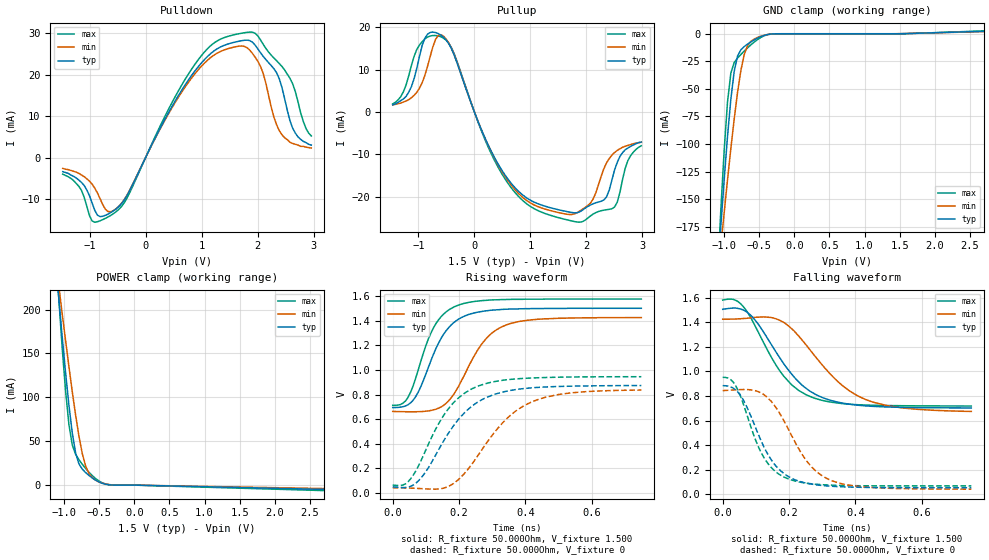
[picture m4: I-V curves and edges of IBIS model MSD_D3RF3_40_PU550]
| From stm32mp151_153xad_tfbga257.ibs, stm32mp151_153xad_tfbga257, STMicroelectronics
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[Model] MSD_D3RF3_40_PU550
Model_type   I/O
C_comp 2.417pF   2.334pF   2.540pF
Vinh = 925.000mV
Vinl = 575.000mV
Vmeas = 750.000mV
Vref = 750.000mV
[Model Spec]
Vinh   925.000mV   888.000mV   963.000mV
Vinl   575.000mV   538.000mV   613.000mV
Vmeas   750.000mV   713.000mV   788.000mV
Vref   750.000mV   713.000mV   788.000mV
[Temperature Range]   25.000   125.000   -40.000
[Voltage Range]   1.500V   1.425V   1.575V
[GND Clamp Reference]   0.00V   0.00V   0.00V
[Pulldown Reference]   0.00V   0.00V   0.00V
[POWER Clamp Reference]   1.500V   1.425V   1.575V
[Pullup Reference]   1.500V   1.425V   1.575V
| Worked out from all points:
|   slope of the pulldown table from 0 to 0.225 V, typ, clamps not added: 36.6 ohm
|   slope of the pullup table from 0 to 0.225 V, typ, clamps not added: 31.2 ohm
|   GND clamp passes 1 mA (typ) near -0.40 V on its own axis
|   POWER clamp passes 1 mA (typ) near -0.41 V on its own axis
|   rising waveform, R_fixture 50.000Ohm, V_fixture 1.500: 20-80 % time 84.3ps typ, 101ps min, 73.8ps max; typ from 0.694 V to 1.5 V
|   rising waveform, R_fixture 50.000Ohm, V_fixture 0: 20-80 % time 131ps typ, 148ps min, 115ps max; typ from 0.05 V to 0.873 V
|   falling waveform, R_fixture 50.000Ohm, V_fixture 1.500: 20-80 % time 134ps typ, 159ps min, 118ps max; typ from 1.5 V to 0.703 V
|   falling waveform, R_fixture 50.000Ohm, V_fixture 0: 20-80 % time 92.7ps typ, 110ps min, 81.1ps max; typ from 0.884 V to 0.055 V
[GND Clamp]
-1.48V    -594.8mA   -480.5mA   -764.4mA
-1.098V   -218.8mA   -223.8mA   -221mA
-1.05V    -174.6mA   -192.8mA   -160.3mA
-1.002V   -132.4mA   -162.4mA   -105.9mA
-954.6mV  -93.29mA   -132.7mA   -62.13mA
-906.8mV  -59.43mA   -104.2mA   -35.7mA
-859.1mV  -34.17mA   -77.46mA   -26.12mA
-811.4mV  -20.23mA   -53.34mA   -22.06mA
-715.9mV  -11.65mA   -18.94mA   -15.73mA
-572.7mV  -5.552mA   -4.746mA   -7.503mA
-286.4mV  -69.21uA   -117uA     -55.41uA
2.959V    2.671mA    2.278mA    3.222mA
[Power Clamp]
-1.459V   578.6mA    480mA      724.3mA
-1.077V   211.6mA    226mA      211.1mA
-1.03V    168.7mA    195.2mA    156.3mA
-981.8mV  128.1mA    164.8mA    107.4mA
-934.1mV  90.98mA    135.1mA    68.88mA
-886.4mV  59.46mA    106.6mA    45.73mA
-838.6mV  36.57mA    79.76mA    35.11mA
-743.2mV  18.16mA    35.82mA    23.68mA
-647.7mV  10.96mA    13.03mA    14.61mA
-552.3mV  5.616mA    5.561mA    7.395mA
-313.6mV  108.4uA    247.8uA    122.3uA
2.98V     -5.382mA   -4.337mA   -6.867mA
[Pulldown]
-1.48V    -3.4mA     -2.6mA     -4mA
-1.145V   -6mA       -4.2mA     -7.9mA
-954.6mV  -10.97mA   -6.4mA     -15.28mA
-715.9mV  -13.9mA    -12.49mA   -14.63mA
-525mV    -12.36mA   -12.29mA   -13.02mA
906.8mV   21.31mA    20.61mA    22.95mA
1.289V    26.28mA    25.22mA    28.18mA
1.766V    28.26mA    26.77mA    30.06mA
2.052V    25.24mA    21.95mA    28.33mA
2.434V    16.91mA    5.5mA      21.96mA
2.625V    7.1mA      3.4mA      17.8mA
2.959V    3mA        2.3mA      5.2mA
[Pullup]
-1.459V   1.7mA      1.7mA      1.929mA
-1.173V   4.7mA      2.929mA    8.571mA
-838.6mV  18.38mA    10.73mA    17.71mA
-695.5mV  18.79mA    17.12mA    18.09mA
-552.3mV  17.7mA     17.94mA    17.47mA
640.9mV   -16.58mA   -16.97mA   -17.62mA
1.834V    -23.79mA   -23.78mA   -25.99mA
2.12V     -21.67mA   -20.55mA   -24.11mA
2.311V    -20.78mA   -13.39mA   -23.19mA
2.502V    -13.7mA    -9.557mA   -22.45mA
2.741V    -8.5mA     -7.886mA   -11.44mA
2.98V     -7.1mA     -7.143mA   -7.971mA
[Ramp]
R_load=50.000Ohm
dV/dt_r   485.190mV/107.500ps  466.302mV/125.500ps  519.564mV/95.000ps
dV/dt_f   485.190mV/113.500ps  466.302mV/137.000ps  519.564mV/100.000ps
[Rising waveform]
R_fixture=50.000Ohm
V_fixture=1.500
V_fixture_min=1.425
V_fixture_max=1.575
0s        694mV      662.5mV    712.1mV
39ps      707.5mV    660.2mV    749.2mV
62ps      755mV      659.9mV    874.2mV
100ps     966.9mV    664.7mV    1.198V
123ps     1.128V     675.3mV    1.342V
154ps     1.292V     713.5mV    1.455V
192ps     1.4V       837.3mV    1.52V
268ps     1.474V     1.209V     1.562V
345ps     1.493V     1.368V     1.572V
749ps     1.5V       1.425V     1.575V
[Rising waveform]
R_fixture=50.000Ohm
V_fixture=0
0s        50.12mV    43.11mV    64.98mV
39ps      45.14mV    41.34mV    75.57mV
77ps      97.7mV     37.26mV    216.8mV
161ps     456.9mV    46.1mV     659.9mV
199ps     600.8mV    111.8mV    774.3mV
245ps     717.8mV    258.9mV    854mV
330ps     819.4mV    567.1mV    915mV
421ps     854.7mV    742.3mV    934.4mV
536ps     867.7mV    812.9mV    942.1mV
749ps     873.1mV    836.5mV    944.6mV
[Falling waveform]
R_fixture=50.000Ohm
V_fixture=1.500
V_fixture_min=1.425
V_fixture_max=1.575
0s        1.505V     1.424V     1.58V
46ps      1.512V     1.427V     1.568V
85ps      1.455V     1.436V     1.434V
177ps     1.09V      1.408V     986.1mV
207ps     981.2mV    1.349V     892.9mV
253ps     859mV      1.209V     808mV
345ps     751.1mV    922.1mV    743.3mV
429ps     720.3mV    773.2mV    727mV
544ps     707.8mV    702.6mV    721.3mV
749ps     703.2mV    674.9mV    718.9mV
[Falling waveform]
R_fixture=50.000Ohm
V_fixture=0
0s        884.2mV    844.3mV    952.3mV
23ps      875.2mV    847.7mV    936.1mV
46ps      831.1mV    851.3mV    847.5mV
69ps      732.3mV    852.8mV    680.7mV
115ps     440mV      825.8mV    344.7mV
154ps     252.6mV    730.6mV    198.3mV
192ps     155.4mV    560.6mV    132.7mV
268ps     83.88mV    223.4mV    86.66mV
337ps     65.49mV    104.2mV    74.99mV
749ps     54.66mV    43.21mV    69.56mV
